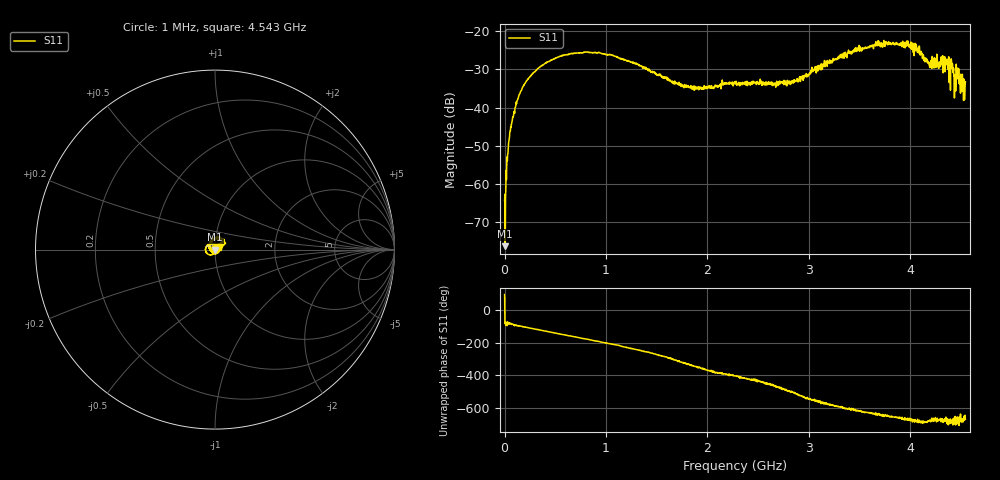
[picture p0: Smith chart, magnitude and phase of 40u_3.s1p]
# HZ S RI R 50
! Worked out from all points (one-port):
!   1515 points, 1 MHz to 4.543 GHz, reference 50 ohm
!   lowest |S11| = -76.4 dB at 7 MHz (marker M1), VSWR 1.00, Z = 50 - j0.0151 ohm
!   |S11| at or under -10 dB: start of sweep to end of sweep
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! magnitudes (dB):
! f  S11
! 1 MHz  -64.4
! 7 MHz  -76.4
! 28 MHz  -54.0
! 37 MHz  -50.8
! 61 MHz  -45.0
! 112 MHz  -39.4
! 160 MHz  -35.7
! 229 MHz  -32.5
! 334 MHz  -29.7
! 571 MHz  -26.3
! 811 MHz  -25.5
! 1.138 GHz  -27.1
! 1.705 GHz  -33.9
! 1.936 GHz  -34.6
! 2.272 GHz  -33.3
! 2.842 GHz  -33.2
! 3.409 GHz  -25.5
! 3.679 GHz  -23.7
! 3.976 GHz  -23.7
! 4.069 GHz  -25.4
! 4.192 GHz  -29.5
! 4.36 GHz  -27.3
! 4.375 GHz  -27.9
! 4.42 GHz  -30.8
! 4.444 GHz  -32.1
! 4.471 GHz  -30.8
! 4.516 GHz  -33.1
! 4.543 GHz  -33.2
